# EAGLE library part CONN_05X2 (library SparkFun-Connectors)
Multi connection point. Often used as Generic Header-pin footprint for 0.1 inch spaced/style header connections For AVR SPI programming port, see special device with nice symbol: "AVR_SPI_PROG_5x2.dev" You can populate with any combo of single row headers, but if you'd like an exact match, check these: 2x5 AVR ICSP Male Header (PRT-00778) 2x5 Pin Shrouded Header (PRT-08506) On any of the 0.1 inch spaced packages, you can populate with these: Break Away Headers - Straight (PRT-00116) Break Away Male Headers - Right Angle (PRT-00553) Female Headers (PRT-00115) Break Away Headers - Machine Pin (PRT-00117) Break Away Female Headers - Swiss Machine Pin (PRT-00743) Special note: the shrouded connector mates well with our 5x2 ribbon cables: 2x5 Pin IDC Ribbon Cable (PRT-08535)
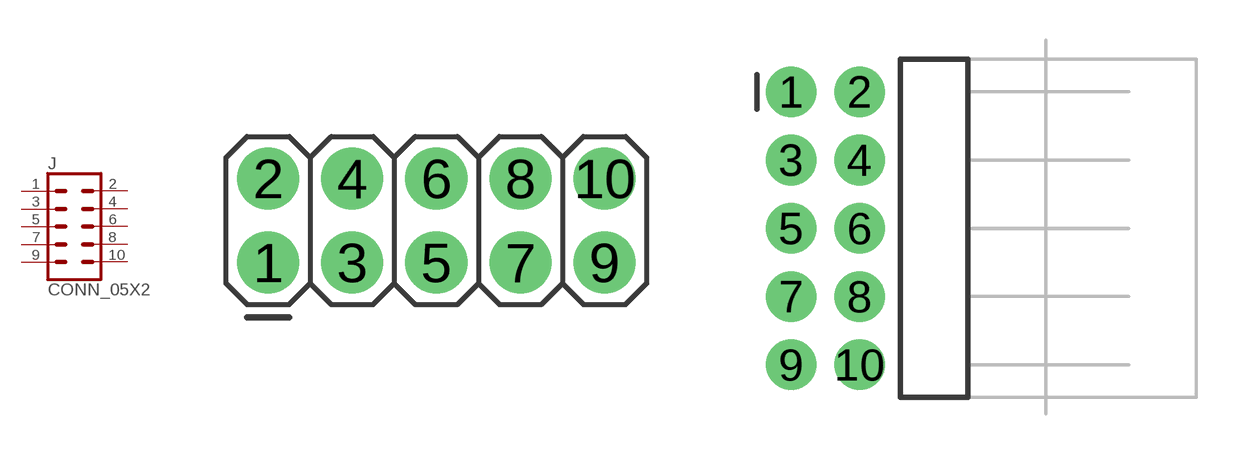
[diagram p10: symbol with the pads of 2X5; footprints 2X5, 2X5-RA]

Designator prefix J

## CONN_05X2PTH (PROD_ID: CONN-08499; SF_ID: PRT-0778)  [2X5]
1  1  pas
2  2  pas
3  3  pas
4  4  pas
5  5  pas
6  6  pas
7  7  pas
8  8  pas
9  9  pas
10  10  pas

## CONN_05X2RA  [2X5-RA]
Pads as for 2X5

## CONN_05X2RAF  [2X5-RAF]
Pads as for 2X5

## CONN_05X2SHD (PROD_ID: CONN-08671; SF_ID: PRT-08506)  [2X5-SHROUDED]
Pads as for 2X5

## CONN_05X2SHD_LOCK (PROD_ID: CONN-08671; SF_ID: PRT-08506)  [2X5-SHROUDED_LOCK]
Pads as for 2X5

## CONN_05X2SHD_SMD (PROD_ID: CONN-09508)  [2X5-SHROUDED_SMD]
Pads as for 2X5

## CONN_05X2NO_SILK  [2X5_NOSILK]
Pads as for 2X5

## CONN_05X20.05_IN_PTH_SILK  [2X5_PTH_SILK_.05]
Pads as for 2X5

## CONN_05X2SHD-NS (PROD_ID: CONN-08671; SF_ID: PRT-08506)  [2X5-SHROUDED-NS]
Pads as for 2X5

## Footprint 2X5 (pad centres in mm)
Plated Through Hole - 2x5 Specifications: Pin count:10 Pin pitch:0.1" Example device(s): CONN_05x2
drill 1.016 pad 1.88: 1 0,0; 2 0,2.54; 3 2.54,0; 4 2.54,2.54; 5 5.08,0; 6 5.08,2.54; 7 7.62,0; 8 7.62,2.54; 9 10.16,0; 10 10.16,2.54

## Footprint 2X5-RA (pad centres in mm)
Plated Through Hole - 2x5 Right Angle Male Headers tDocu shows pin location. Specifications: Pin count:10 Pin pitch:0.1" Example device(s): CONN_05x2
drill 1.016 pad 1.88: 1 -1.27,5.08; 2 1.27,5.08; 3 -1.27,2.54; 4 1.27,2.54; 5 -1.27,0; 6 1.27,0; 7 -1.27,-2.54; 8 1.27,-2.54; 9 -1.27,-5.08; 10 1.27,-5.08

## Footprint 2X5-RAF (pad centres in mm)
Plated Through Hole - 2x5 Right Angle Female Header Silk outline of pins Specifications: Pin count:10 Pin pitch:0.1" Example device(s): CONN_05x2
drill 1.016 pad 1.88: 1 -1.27,5.08; 2 1.27,5.08; 3 -1.27,2.54; 4 1.27,2.54; 5 -1.27,0; 6 1.27,0; 7 -1.27,-2.54; 8 1.27,-2.54; 9 -1.27,-5.08; 10 1.27,-5.08

## Footprint 2X5-SHROUDED (pad centres in mm)
Plated Through Hole - 2x5 Shrouded Header Specifications: Pin count:10 Pin pitch:0.1" Datasheet referenced for footprint Example device(s): CONN_05x2
drill 1.016 pad 1.88: 1 -1.27,5.08; 2 1.27,5.08; 3 -1.27,2.54; 4 1.27,2.54; 5 -1.27,0; 6 1.27,0; 7 -1.27,-2.54; 8 1.27,-2.54; 9 -1.27,-5.08; 10 1.27,-5.08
